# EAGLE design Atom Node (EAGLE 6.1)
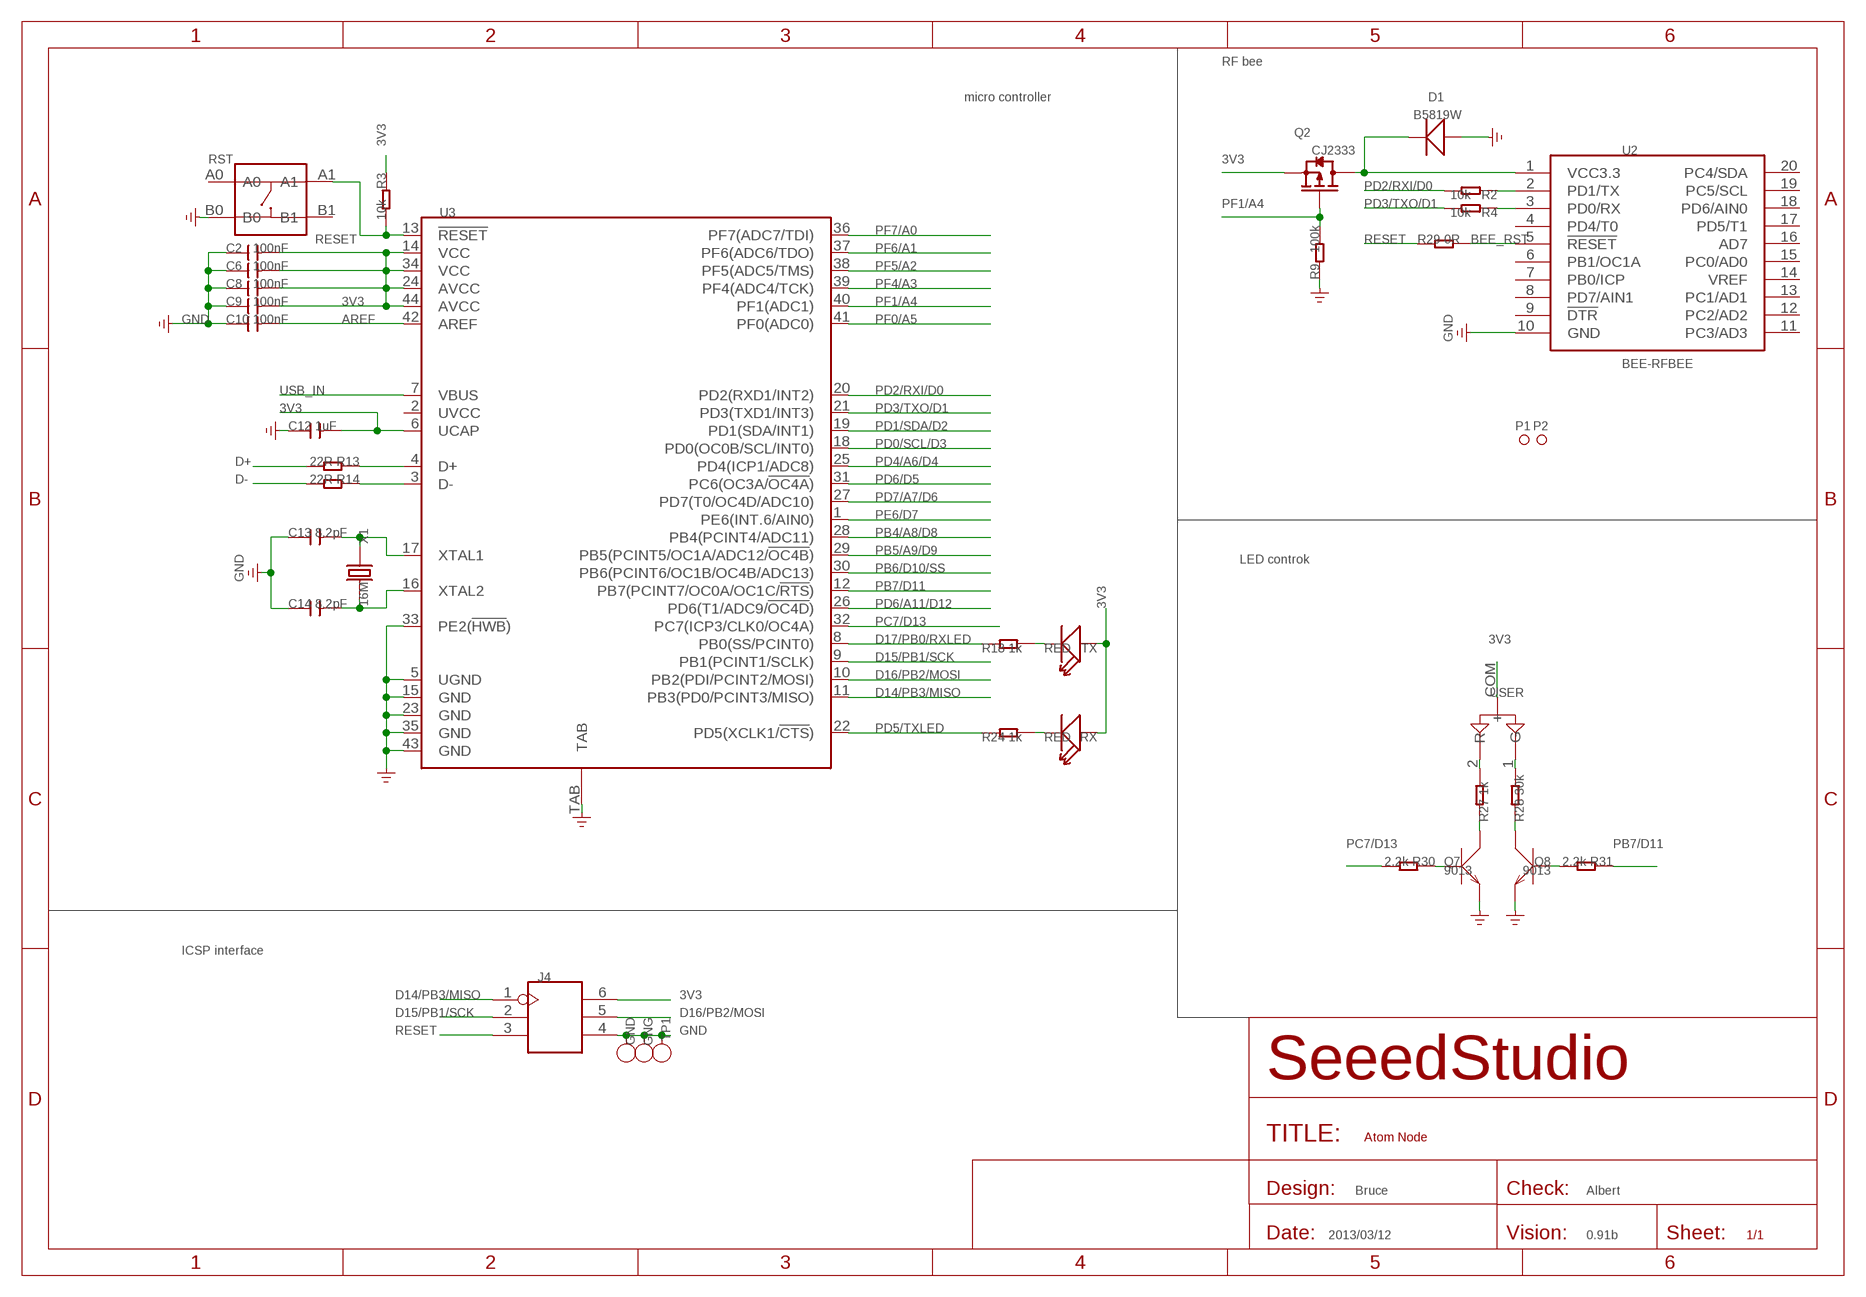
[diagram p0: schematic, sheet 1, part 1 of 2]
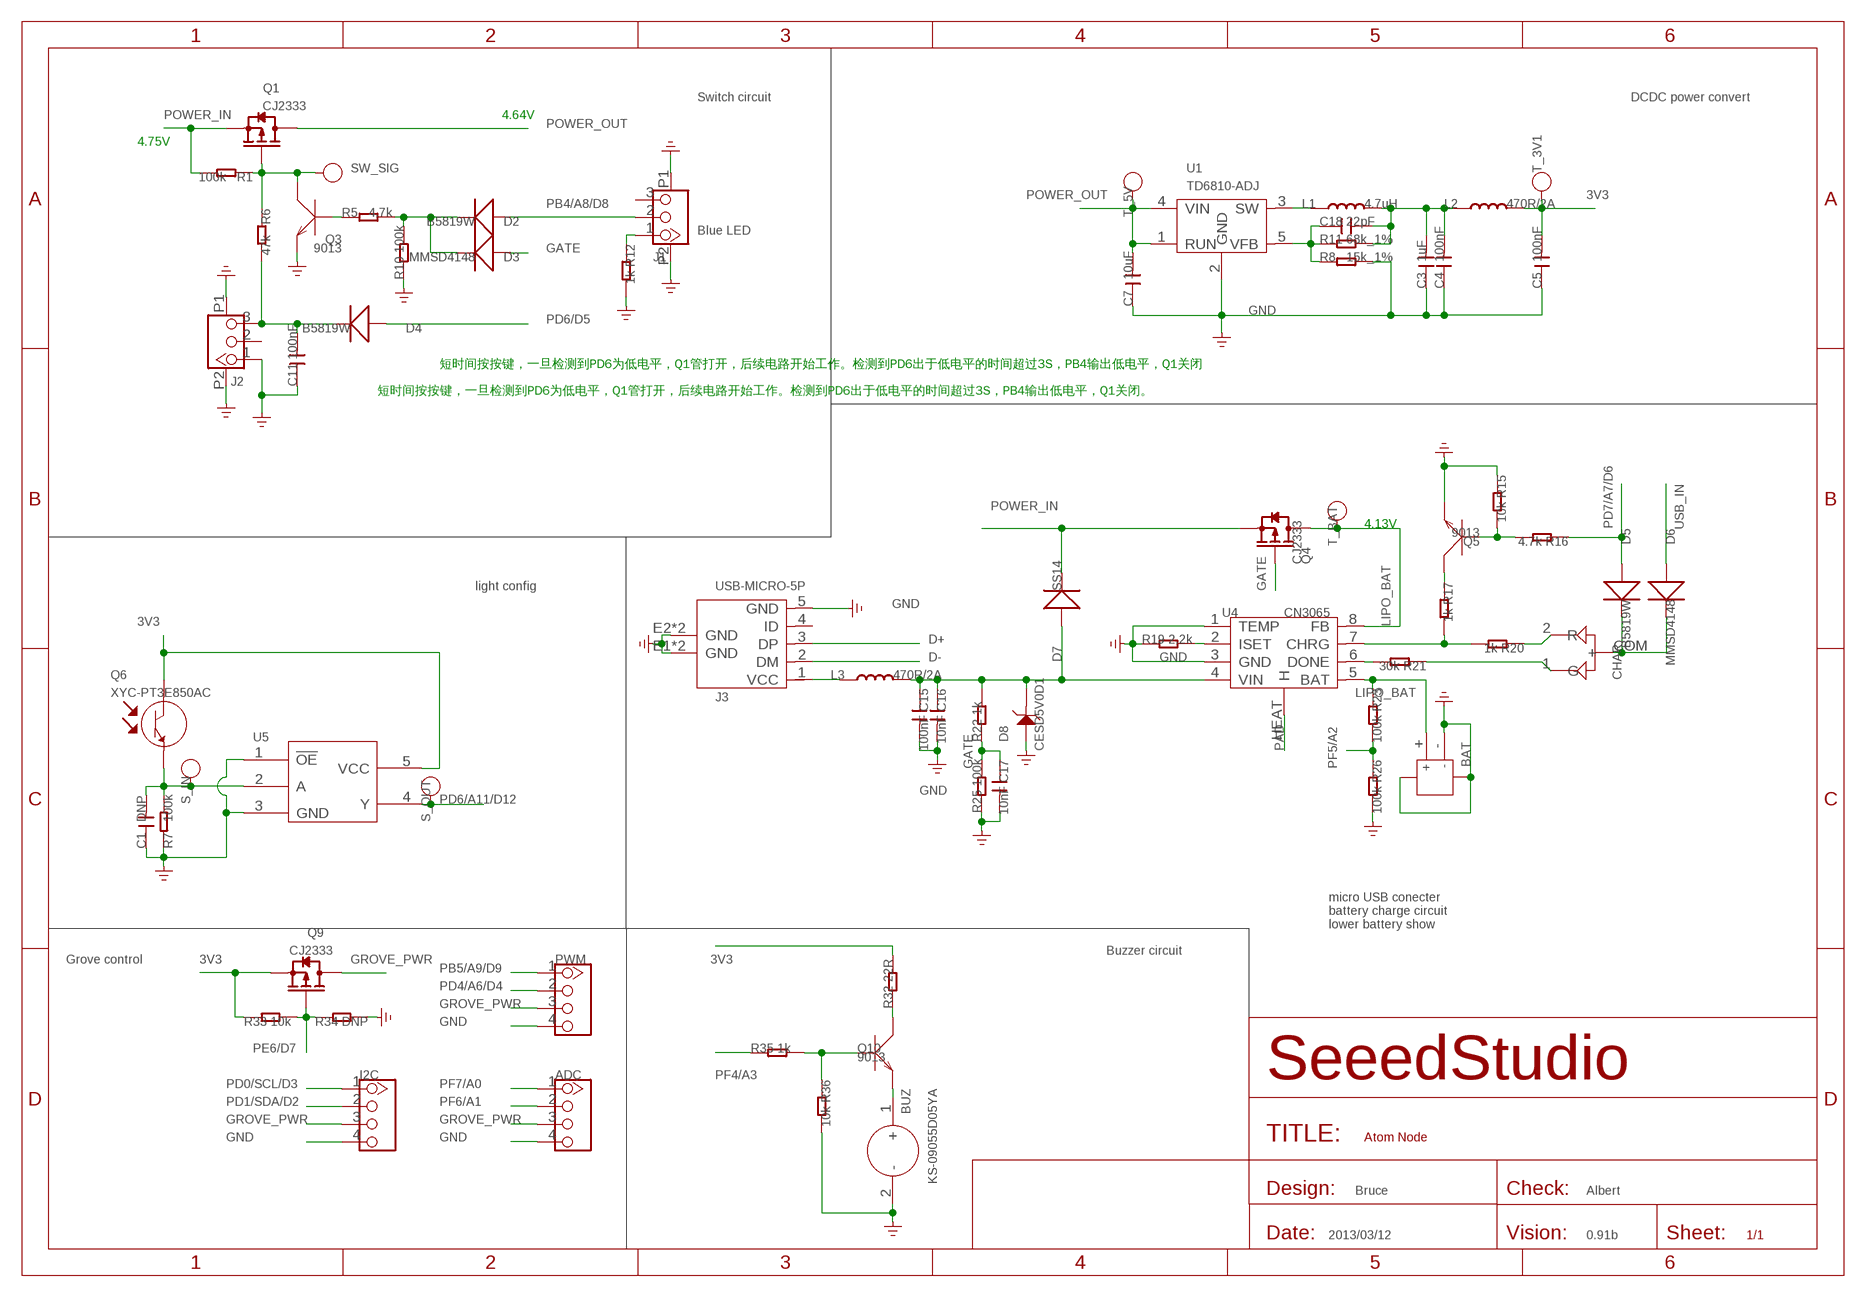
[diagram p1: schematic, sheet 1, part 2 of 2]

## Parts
ADC  TWIG-4P-2.0-2.0  [4P-2.0]
BAT  JACK-JST-2P-SMD-PW'1.0'  [JST-SMD-2P-1.0-90D]
BUZ  KS-09055D05YA  BUZZER-AT0955V5  [2P-5.0-D9.0X5.5H]
C1  DNP  C-0603  [C0603]
C2  100nF  C-0603  [C0603]
C3  1uF  C-0603  [C0603]
C4  100nF  C-0603  [C0603]
C5  100nF  C-0603  [C0603]
C6  100nF  C-0603  [C0603]
C7  10uF  C-0805  [C0805]
C8  100nF  C-0603  [C0603]
C9  100nF  C-0603  [C0603]
C10  100nF  C-0603  [C0603]
C11  100nF  C-0603  [C0603]
C12  1uF  C-0603  [C0603]
C13  8.2pF  C-0603  [C0603]
C14  8.2pF  C-0603  [C0603]
C15  100nF  C-0603  [C0603]
C16  10nF  C-0603  [C0603]
C17  10nF  C-0603  [C0603]
C18  22pF  C-0603  [C0603]
CHAR  LED-ARG-3P'-3MM'  [LED-3P-2.54-3MM]
D1  B5819W  D'1206'  [SOD123]
D2  B5819W  D'1206'  [SOD123]
D3  MMSD4148  D'1206'  [SOD123]
D4  B5819W  D'1206'  [SOD123]
D5  B5819W  D'1206'  [SOD123]
D6  MMSD4148  D'1206'  [SOD123]
D7  SS14  D'B130L-13-F'  [SMA]
D8  CESD5V0D1  D-ESD-2P'CESD5V0D1'  [SOD123-2.7X1.6]
GND  PAD-TEST-POINT-CIRCLE'4545'  [TP_4545]
GNG  PAD-TEST-POINT-CIRCLE'4545'  [TP_4545]
I2C  TWIG-4P-2.0-2.0  [4P-2.0]
J1  JST-3P-1.0  [3P-SMD-1.0]
J2  JST-3P-1.0  [3P-SMD-1.0]
J3  USB-MICRO-5P  [MICRO-USB-5P]
J4  HEADER-2X3P-2.0  [2X3P-2.0]
L1  4.7uH  LSPD3D16-4R7M  [L0420]
L2  470R/2A  L'0805'  [L0805]
L3  470R/2A  L'0805'  [L0805]
P1  PAD-MARK  [ROUND-MARK-1.0]
P2  PAD-MARK  [ROUND-MARK-1.0]
PWM  TWIG-4P-2.0-2.0  [4P-2.0]
Q1  CJ2333  MOSFET-P'SI2323CDS/SI2305DS<BR>'  [SOT23]
Q2  CJ2333  MOSFET-P'SI2323CDS/SI2305DS<BR>'  [SOT23]
Q3  9013  TRANSISTOR-NPN-SOT23  [SOT23]
Q4  CJ2333  MOSFET-P'SI2323CDS/SI2305DS<BR>'  [SOT23]
Q5  9013  TRANSISTOR-NPN-SOT23  [SOT23]
Q6  XYC-PT3E850AC  PHOTISTOR-PT550'XYC-PT3E550AC-IC'  [2P-D3MMX3.85H]
Q7  9013  TRANSISTOR-NPN-SOT23  [SOT23]
Q8  9013  TRANSISTOR-NPN-SOT23  [SOT23]
Q9  CJ2333  MOSFET-P'SI2323CDS/SI2305DS<BR>'  [SOT23]
Q10  9013  TRANSISTOR-NPN-SOT23  [SOT23]
R1  100k  R-0603  [R0603]
R2  10k  R-0603  [R0603]
R3  10k  R-0603  [R0603]
R4  10k  R-0603  [R0603]
R5  4.7k  R-0603  [R0603]
R6  47k  R-0603  [R0603]
R7  100k  R-0603  [R0603]
R8  15k_1%  R-0603  [R0603]
R9  100k  R-0603  [R0603]
R10  100k  R-0603  [R0603]
R11  68k_1%  R-0603  [R0603]
R12  1k  R-0603  [R0603]
R13  22R  R-0603  [R0603]
R14  22R  R-0603  [R0603]
R15  10k  R-0603  [R0603]
R16  4.7k  R-0603  [R0603]
R17  1k  R-0603  [R0603]
R18  1k  R-0603  [R0603]
R19  2.2k  R-0603  [R0603]
R20  1k  R-0603  [R0603]
R21  30k  R-0603  [R0603]
R22  1k  R-0603  [R0603]
R23  100k  R-0603  [R0603]
R24  1k  R-0603  [R0603]
R25  100k  R-0603  [R0603]
R26  100k  R-0603  [R0603]
R27  1k  R-0603  [R0603]
R28  30k  R-0603  [R0603]
R29  0R  R-0603  [R0603]
R30  2.2k  R-0603  [R0603]
R31  2.2k  R-0603  [R0603]
R32  22R  R-0603  [R0603]
R33  10k  R-0603  [R0603]
R34  DNP  R-0603  [R0603]
R35  1k  R-0603  [R0603]
R36  10k  R-0603  [R0603]
RST  BUTTON-4P-3.3X3.3  [4P-SMD-3.4X3.4X1.3H]
RX  RED  LED'0603'  [LED-0603]
S_IN  PAD-TEST-POINT-CIRCLE'4545'  [TP_4545]
S_OUT  PAD-TEST-POINT-CIRCLE'4545'  [TP_4545]
SW_SIG  PAD-TEST-POINT-CIRCLE'4545'  [TP_4545]
T_3V1  PAD-TEST-POINT-CIRCLE'4545'  [TP_4545]
T_5V  PAD-TEST-POINT-CIRCLE'4545'  [TP_4545]
T_BAT  PAD-TEST-POINT-CIRCLE'4545'  [TP_4545]
TP1  PAD-TEST-POINT-CIRCLE'4545'  [TP_4545]
TX  RED  LED'0603'  [LED-0603]
U1  TD6810-ADJ  TD6810'TSOT23-5'  [SOT23-5]
U2  BEE-RFBEE  [20P-DIP-2.0-PRO]
U3  ATMEGA32U4-QFN44  [QFN44]
U4  CN3065  [DFN8]
U5  74AUP1G17GW  SN74LVC1G125DCKR  [SOT353]
USER  LED-ARG-3P'-3MM'  [LED-3P-2.54-3MM]
X1  16M  CRYSTAL'5032'  [2P-SMD-5X3.2]

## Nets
3V3: C2.2 C5.2 C6.2 C8.2 C9.2 C12.2 J4.6 L2.2 Q2.2(S) Q6.C Q9.2(S) R3.1 R32.2 R33.1 RX.+ T_3V1.T TX.+ U3.6(UCAP) U3.14(VCC) U3.24(AVCC) U3.34(VCC) U3.44(AVCC) U5.5(VCC) USER.COM(+)
AREF: C10.2 U3.42(AREF)
BEE_RST: R29.2 U2.5(!RESET)
D14/PB3/MISO: J4.1 U3.11(PB3(PD0/PCINT3/MISO))
D15/PB1/SCK: J4.2 U3.9(PB1(PCINT1/SCLK))
D16/PB2/MOSI: J4.5 U3.10(PB2(PDI/PCINT2/MOSI))
D17/PB0/RXLED: R18.1 U3.8(PB0(SS/PCINT0))
D+: J3.3(DP) R13.2
D-: J3.2(DM) R14.2
GATE: C17.1 D3.+ Q4.1(G) R22.1 R25.2
GND: ADC.4 BAT.3 BAT.4 BAT.- BUZ.2(-) C1.1 C2.1 C3.1 C4.1 C5.1 C6.1 C7.1 C8.1 C9.1 C10.1 C11.1 C12.1 C13.1 C14.1 C15.2 C16.2 C17.2 D1.+ D8.1 GND.T GNG.T I2C.4 J1.P1 J1.P2 J2.1 J2.P1 J2.P2 J3.5(GND) J3.E1(GND) J3.E2(GND) J3.P1(GND) J3.P2(GND) J4.4 PWM.4 Q3.2(E) Q5.2(E) Q7.2(E) Q8.2(E) R7.1 R8.2 R9.1 R10.1 R12.2 R15.1 R19.1 R25.1 R26.2 R34.2 R36.2 RST.B0 TP1.T U1.2(GND) U2.10(GND) U3.5(UGND) U3.15(GND) U3.23(GND) U3.33(PE2(!HWB!)) U3.35(GND) U3.43(GND) U3.TAB U4.1(TEMP) U4.3(GND) U5.1(!OE!) U5.3(GND)
GROVE_PWR: ADC.3 I2C.3 PWM.3 Q9.3(D)
LIPO_BAT: BAT.+ Q4.3(D) R23.1 T_BAT.T U4.5(BAT) U4.8(FB)
N$1: CHAR.COM(+) D5.- D6.-
N$2: Q5.3(C) R17.1
N$3: Q10.3(C) R32.1
N$4: C1.2 Q6.E R7.2 S_IN.T U5.2(A)
N$5: C11.2 D4.- J2.3 R6.2
N$6: BUZ.1(+) Q10.2(E)
N$7: R19.2 U4.2(ISET)
N$8: R17.2 R20.2 U4.7(CHRG)
N$9: R21.2 U4.6(DONE)
N$10: Q1.1(G) Q3.3(C) R1.1 R6.1 SW_SIG.T
N$11: Q10.1(B) R35.2 R36.1
N$12: Q3.1(B) R5.1
N$13: D2.- D3.- R5.2 R10.2
N$14: J3.1(VCC) L3.1
N$15: D1.- Q2.3(D) U2.1(VCC3.3)
N$16: R2.1 U2.2(PD1/TX)
N$17: R4.1 U2.3(PD0/RX)
N$26: Q5.1(B) R15.2 R16.2
N$27: J1.1 R12.1
N$29: L1.1 U1.3(SW)
N$31: C13.2 U3.17(XTAL1) X1.1
N$32: C14.2 U3.16(XTAL2) X1.2
N$33: R18.2 TX.-
N$34: R24.2 RX.-
N$35: Q7.1(B) R30.1
N$37: R13.1 U3.4(D+)
N$38: R14.1 U3.3(D-)
N$39: C18.1 R8.1 R11.1 U1.5(VFB)
N$40: R27.2 USER.2(R)
N$41: CHAR.2(R) R20.1
N$42: CHAR.1(G) R21.1
N$43: R28.2 USER.1(G)
N$44: Q7.3(C) R27.1
N$45: Q8.3(C) R28.1
N$46: Q8.1(B) R31.2
N$47: C3.2 C4.2 C18.2 L1.2 L2.1 R11.2
PAD: U4.HEAT(H)
PB4/A8/D8: D2.+ J1.2 U3.28(PB4(PCINT4/ADC11))
PB5/A9/D9: PWM.1 U3.29(PB5(PCINT5/OC1A/ADC12/!OC4B!))
PB6/D10/SS: U3.30(PB6(PCINT6/OC1B/OC4B/ADC13))
PB7/D11: R31.1 U3.12(PB7(PCINT7/OC0A/OC1C/!RTS!))
PC7/D13: R30.2 U3.32(PC7(ICP3/CLK0/OC4A))
PD0/SCL/D3: I2C.1 U3.18(PD0(OC0B/SCL/INT0))
PD1/SDA/D2: I2C.2 U3.19(PD1(SDA/INT1))
PD2/RXI/D0: R2.2 U3.20(PD2(RXD1/INT2))
PD3/TXO/D1: R4.2 U3.21(PD3(TXD1/INT3))
PD4/A6/D4: PWM.2 U3.25(PD4(ICP1/ADC8))
PD5/TXLED: R24.1 U3.22(PD5(XCLK1/!CTS!))
PD6/A11/D12: S_OUT.T U3.26(PD6(T1/ADC9/!OC4D!)) U5.4(Y)
PD6/D5: D4.+ U3.31(PC6(OC3A/!OC4A!))
PD7/A7/D6: D5.+ R16.1 U3.27(PD7(T0/OC4D/ADC10))
PE6/D7: Q9.1(G) R33.2 R34.1 U3.1(PE6(INT.6/AIN0))
PF0/A5: U3.41(PF0(ADC0))
PF1/A4: Q2.1(G) R9.2 U3.40(PF1(ADC1))
PF4/A3: R35.1 U3.39(PF4(ADC4/TCK))
PF5/A2: R23.2 R26.1 U3.38(PF5(ADC5/TMS))
PF6/A1: ADC.2 U3.37(PF6(ADC6/TDO))
PF7/A0: ADC.1 U3.36(PF7(ADC7/TDI))
POWER_IN: D7.1(-) Q1.2(S) Q4.2(S) R1.2
POWER_OUT: C7.2 Q1.3(D) T_5V.T U1.1(RUN) U1.4(VIN)
RESET: J4.3 R3.2 R29.1 RST.A1 U3.13(!RESET)
USB_IN: C15.1 C16.1 D6.+ D7.2(+) D8.2 L3.2 R22.2 U3.7(VBUS) U4.4(VIN)
Unconnected: J1.3 J2.2 J3.4(ID) RST.A0 RST.B1 U2.4(PD4/T0) U2.6(PB1/OC1A) U2.7(PB0/ICP) U2.8(PD7/AIN1) U2.9(!DTR) U2.11(PC3/AD3) U2.12(PC2/AD2) U2.13(PC1/AD1) U2.14(VREF) U2.15(PC0/AD0) U2.16(AD7) U2.17(PD5/T1) U2.18(PD6/AIN0) U2.19(PC5/SCL) U2.20(PC4/SDA) U3.2(UVCC)

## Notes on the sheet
- RF bee
- micro controller | Switch circuit | DCDC power convert
- 4.64V
- 4.75V
- Blue LED
- 短时间按按键，一旦检测到PD6为低电平，Q1管打开，后续电路开始工作。检测到PD6出于低电平的时间超过3S，PB4输出低电平，Q1关闭
- 短时间按按键，一旦检测到PD6为低电平，Q1管打开，后续电路开始工作。检测到PD6出于低电平的时间超过3S，PB4输出低电平，Q1关闭。
- 4.13V
- LED controk
- light config
- micro USB conecter
  battery charge circuit
  lower battery show
- ICSP interface | Buzzer circuit
- Grove control
- Bruce | Albert | Bruce | Albert
- 2013/03/12 | 0.91b | 2013/03/12 | 0.91b

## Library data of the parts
ADC I2C PWM = Connector:TWIG-4P-2.0
BAT = Connector:JACK-JST-2P-SMD-PW
BUZ = Discrete:BUZZER
C1-C18 = Discrete:C*: Ceramic Capacitors
CHAR USER = Discrete:LED-ARG-3P
D1-D7 = Discrete:D*
D8 = Discrete:D-ESD-2P: Diodes for Protectiong against ESD
GND GNG S_IN S_OUT SW_SIG T_3V1 T_5V T_BAT TP1 = Discrete:PAD-TEST-POINT-CIRCLE; PARTNO: DNP
J1 J2 = template:JST-3P-1.0
J3 = Connector:USB-MICRO-5P
J4 = Connector:HEADER-2X3P
L1 = template:L
L2 L3 = Discrete:L*
P1 P2 = Discrete:PAD-MARK; PARTNO: DNP
Q1 Q2 Q4 Q9 = Discrete:MOSFET-P
Q3 Q5 Q7 Q8 Q10 = Discrete:TRANSISTOR-NPN*: NPN audion
Q6 = template:PHOTISTOR-PT550
R1-R36 = Discrete:R*
RST = Discrete:BUTTON-4P
RX TX = Discrete:LED*
U1 = template:TD6810: 1.5MHz 800mA Synchronous Step-Down Regulator Dropout http://www.techcodeok.com/download/TD6810.pdf
U2 = moudle:BEE-RFBEE
U3 = IC:ATMEGA32U4-QFN44: 8-bit Microcontroller With 16/32K Bytes of ISP Flash and USB controller
U4 = IC:CN3065
U5 = template:SN74LVC1G125DCKR: Signal bus buffer gate
X1 = Discrete:CRYSTAL*: CRYSTAL

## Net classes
0 default: width 0.152 mm, drill 0.305 mm, clearance 0.152 mm
3 none3: width 0.203 mm, drill 0.305 mm, clearance 0.203 mm

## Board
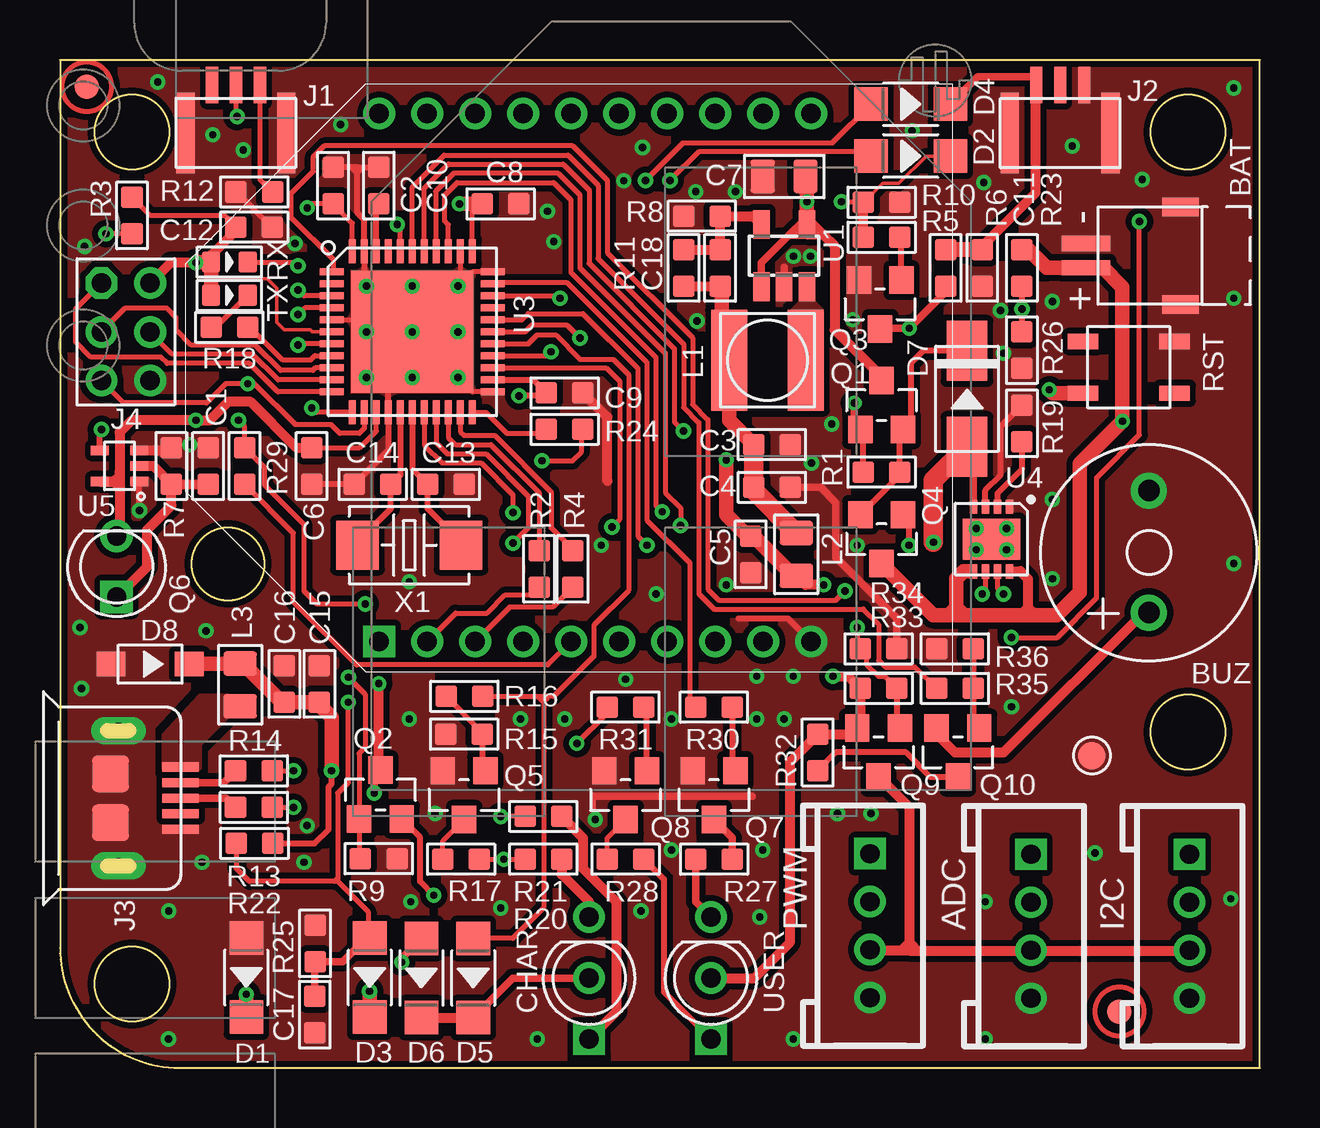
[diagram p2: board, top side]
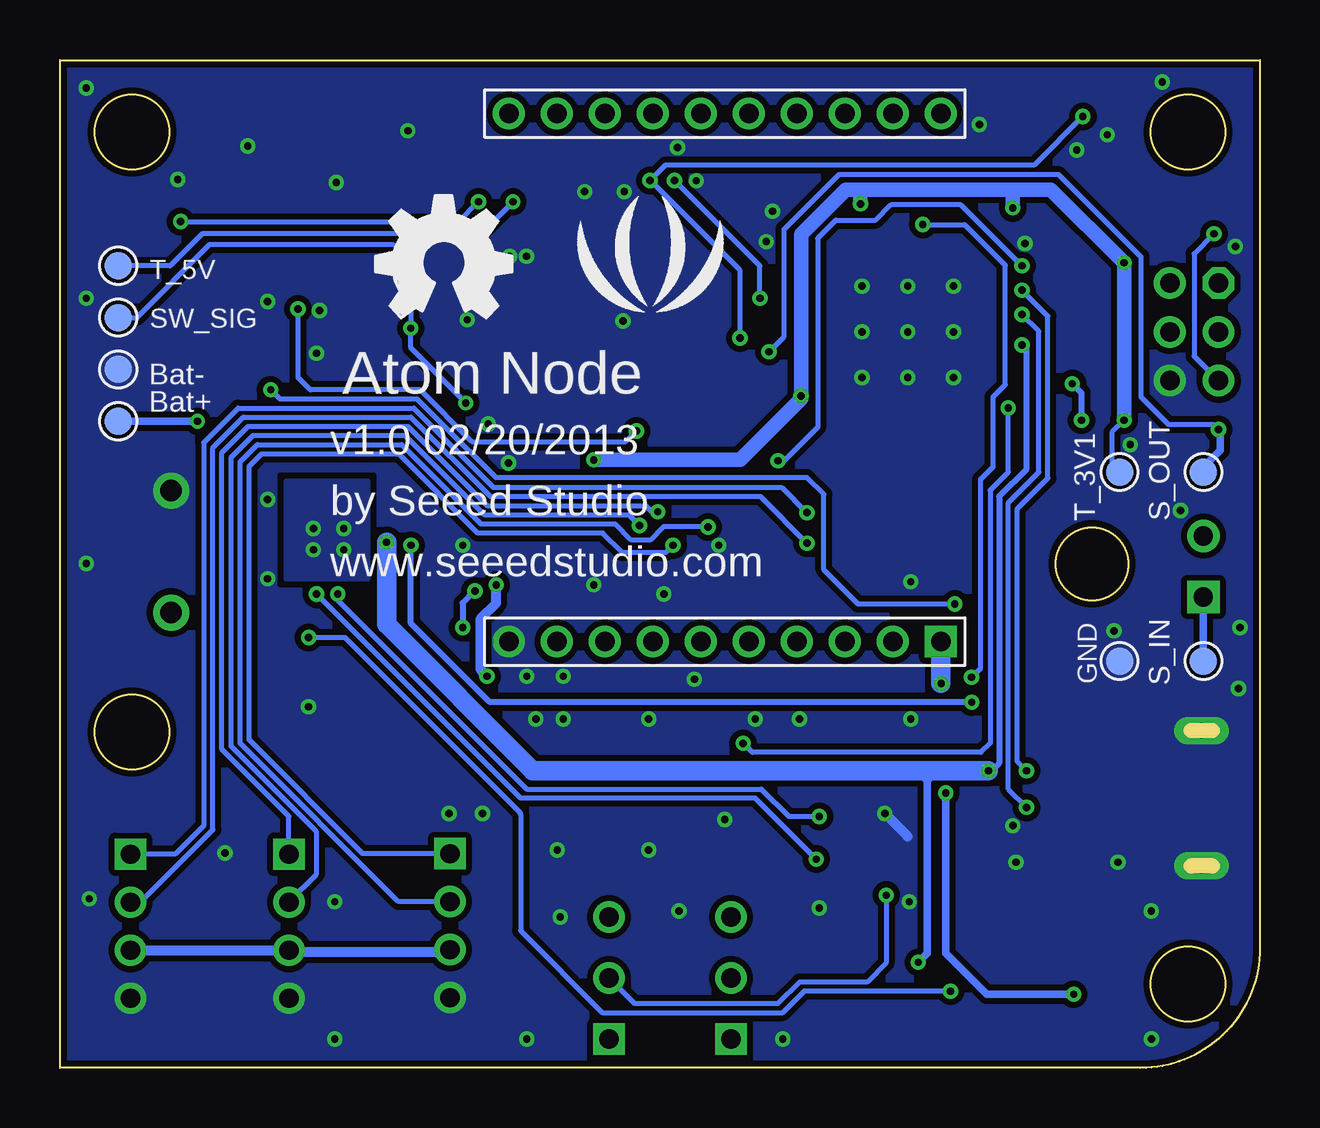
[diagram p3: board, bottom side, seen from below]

Size 50 x 42 mm. Coordinates in mm from the lower left corner, seen from the top.
Outline: 5,0 4.76,0 4.52,0.02 4.29,0.05 4.05,0.09 3.82,0.14 3.59,0.2 3.36,0.27 3.14,0.36 2.92,0.45 2.71,0.56 2.5,0.67 2.3,0.79 2.1,0.93 1.91,1.07 1.72,1.22 1.55,1.38 1.38,1.55 1.22,1.72 1.07,1.91 0.93,2.1 0.79,2.3 0.67,2.5 0.56,2.71 0.45,2.92 0.36,3.14 0.27,3.36 0.2,3.59 0.14,3.82 0.09,4.05 0.05,4.29 0.02,4.52 0.01,4.76 0,5 0,42 50,42 50,0 5,0
Outline: circle at 3,39 radius 1.55
Outline: circle at 7,21 radius 1.52
Outline: circle at 47,39 radius 1.55
Outline: circle at 3,3.5 radius 1.55
Outline: circle at 47,14 radius 1.55
Copper layers (1*16): Top 0.035mm / dielectric 1.5mm / Bottom 0.035mm
Design rules "SeeedStudio_rule_no_angle_090911 *": minimum track width 6mil, minimum drill 12mil, track to track 6mil, track to pad 6mil, pad to pad 6mil, via to via 6mil, smd to smd 0mil, copper to edge 8mil, drill to drill 10mil, minimum pad ring 10mil, minimum via ring 6mil, stop-mask expansion 2mil, vias tented up to drill 25mil, thermal gap 10mil
tRestrict: area 28,27.4 to 30.9,31.4

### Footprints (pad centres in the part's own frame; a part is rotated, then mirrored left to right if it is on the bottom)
4P-2.0 = drill 0.8 pad 1.27 square: 1 -3,0 | drill 0.8 pad 1.27: 2 -1,0; 3 1,0; 4 3,0
JST-SMD-2P-1.0-90D = smd 1.524 x 0.762: 3 -3.429,2.032; 4 -3.429,-2.032 | smd 2.032 x 0.635: + 0.508,0.508; - 0.508,-0.508
2P-5.0-D9.0X5.5H = drill 0.9 pad 1.5: 1 -2.5,0; 2 2.58,0
C0603 = smd 0.889 x 0.889: 1 -0.762,0; 2 0.762,0
C0805 = smd 1.016 x 1.397: 1 -0.889,0; 2 0.889,0
LED-3P-2.54-3MM = drill 0.8 pad 1.3 square: 1 -2.54,0 | drill 0.8 pad 1.3: 2 2.54,0; COM 0,0
SOD123 = smd 1.397 x 1.397: + -1.651,0; - 1.651,0
SMA = smd 2.5 x 1.7: 1 2,0; 2 -2,0
SOD123-2.7X1.6 = smd 1.2 x 1.02: 1 -1.635,0; 2 1.635,0
TP_4545 = smd 1.143 x 1.143: T 0,0
3P-SMD-1.0 = smd 1.524 x 0.508: 1 -2,1; 2 -2,0; 3 -2,-1 | smd 3.353 x 0.762: P1 0,-2.1; P2 0,2.1
MICRO-USB-5P = smd 0.38 x 1.52: 1 -1.3,0; 2 -0.65,0; 3 0,0; 4 0.65,0; 5 1.3,0 | smd 1.524 x 1.524: E1 -1.016,-2.921; E2 1.016,-2.921 | drill 0.635 pad 1.143 long: P1 -2.819,-2.591; P2 2.819,-2.591
2X3P-2.0 = drill 0.813 pad 1.27 octagon: 1 -1.016,2.032 | drill 0.813 pad 1.27: 2 -1.016,0; 3 -1.016,-2.032; 4 1.016,-2.032; 5 1.016,0; 6 1.016,2.032
L0420 = smd 1.5 x 4.2: 1 -1.6,0; 2 1.6,0
L0805 = smd 1.016 x 1.397: 1 -0.889,0; 2 0.889,0
ROUND-MARK-1.0 = smd 1.016 x 1.016: P$1 0,0
SOT23 = smd 1.016 x 1.143: 1 -0.889,-1.016; 2 0.889,-1.016; 3 0,1.016
2P-D3MMX3.85H = drill 0.8 pad 1.35: C 1.27,0 | drill 0.8 pad 1.35 square: E -1.27,0
R0603 = smd 0.889 x 0.889: 1 -0.762,0; 2 0.762,0
4P-SMD-3.4X3.4X1.3H = smd 1.27 x 0.635: A0 -1.905,1.079; A1 1.905,1.079; B0 -1.905,-1.079; B1 1.905,-1.079
LED-0603 = smd 0.762 x 0.889: + -0.762,0; - 0.762,0
SOT23-5 = smd 0.69 x 1.2: 1 -0.95,-1.3; 2 0,-1.3; 3 0.95,-1.3; 4 0.95,1.3; 5 -0.95,1.3
20P-DIP-2.0-PRO = drill 0.813 square: 1 -11,9 | drill 0.813: 2 -11,7; 3 -11,5; 4 -11,3; 5 -11,1; 6 -11,-1; 7 -11,-3; 8 -11,-5; 9 -11,-7; 10 -11,-9; 11 11,-9; 12 11,-7; 13 11,-5; 14 11,-3; 15 11,-1; 16 11,1; 17 11,3; 18 11,5; 19 11,7; 20 11,9
QFN44 = smd 1 x 0.3: 1 -3.35,2.5; 2 -3.35,2; 3 -3.35,1.5; 4 -3.35,1; 5 -3.35,0.5; 6 -3.35,0; 7 -3.35,-0.5; 8 -3.35,-1; 9 -3.35,-1.5; 10 -3.35,-2; 11 -3.35,-2.5; 23 3.35,-2.5; 24 3.35,-2; 25 3.35,-1.5; 26 3.35,-1; 27 3.35,-0.5; 28 3.35,0; 29 3.35,0.5; 30 3.35,1; 31 3.35,1.5; 32 3.35,2; 33 3.35,2.5 | smd 0.3 x 1: 12 -2.5,-3.35; 13 -2,-3.35; 14 -1.5,-3.35; 15 -1,-3.35; 16 -0.5,-3.35; 17 0,-3.35; 18 0.5,-3.35; 19 1,-3.35; 20 1.5,-3.35; 21 2,-3.35; 22 2.5,-3.35; 34 2.5,3.35; 35 2,3.35; 36 1.5,3.35; 37 1,3.35; 38 0.5,3.35; 39 0,3.35; 40 -0.5,3.35; 41 -1,3.35; 42 -1.5,3.35; 43 -2,3.35; 44 -2.5,3.35 | smd 5.08 x 5.08: TAB 0,0
DFN8 = smd 0.3 x 0.6: 1 -0.75,-1.35; 2 -0.25,-1.35; 3 0.25,-1.35; 4 0.75,-1.35; 5 0.75,1.35; 6 0.25,1.35; 7 -0.25,1.35; 8 -0.75,1.35 | smd 2.4 x 1.7: HEAT 0,0
SOT353 = smd 0.4 x 0.75: 1 -0.65,-0.825; 2 0,-0.825; 3 0.65,-0.825; 4 0.65,0.825; 5 -0.65,0.825
2P-SMD-5X3.2 = smd 1.778 x 2.032: 1 -2.159,0; 2 2.159,0

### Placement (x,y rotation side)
ADC  40.46,5.91 270 top
BAT  43.25,33.85 180 top
BUZ  45.37,21.48 90 top
C1  6.17,25.08 270 top
C2  11.38,36.77 270 top
C3  29.66,25.97 180 top
C4  29.66,24.19 180 top
C5  28.78,21.4 90 top
C6  10.49,25.08 90 top
C7  30.17,37.15 0 top
C8  18.36,36.01 180 top
C9  21.03,28.13 180 top
C10  13.28,36.77 270 top
C11  38.43,33.34 90 top
C12  8.09,35.04 180 top
C13  16.08,24.32 180 top
C14  13.03,24.32 0 top
C15  10.8,16 90 top
C16  9.34,16 90 top
C17  10.61,2.22 270 top
C18  27.51,33.34 270 top
CHAR  22.04,3.75 90 top
D1  7.76,3.77 270 top
D2  35.45,38 0 top
D3  12.91,3.77 270 top
D4  35.45,40.16 0 top
D5  17.22,3.75 270 top
D6  15.06,3.75 270 top
D7  37.79,27.88 90 top
D8  3.76,16.83 0 top
GND  5.85,16.96 90 bottom
GNG  43,13.02 270 top
I2C  47.06,5.91 270 top
J1  7.33,38.96 270 top
J2  41.67,38.95 270 top
J3  5.03,11.24 270 top
J4  2.74,30.67 0 top
L1  29.48,29.49 180 top
L2  30.68,21.4 270 top
L3  7.51,15.96 90 top
P1  1.11,40.88 270 top
P2  44.14,2.35 270 top
PWM  33.75,5.93 270 top
Q1  34.24,27.62 0 top
Q2  13.35,11.39 0 top
Q3  34.17,31.81 180 top
Q4  34.24,22.04 180 top
Q5  16.84,11.37 180 top
Q6  2.36,20.89 90 top
Q7  27.25,11.37 180 top
Q8  23.57,11.37 180 top
Q9  34.11,13.15 180 top
Q10  37.41,13.15 180 top
R1  34.24,24.83 0 top
R2  19.96,20.79 90 top
R3  3,35.52 270 top
R4  21.36,20.79 90 top
R5  34.24,34.61 180 top
R6  36.9,33.34 90 top
R7  4.65,25.08 270 top
R8  26.74,35.5 180 top
R9  13.28,8.72 180 top
R10  34.24,36.07 180 top
R11  25.98,33.34 270 top
R12  8.09,36.5 180 top
R13  8.07,10.86 180 top
R14  8.07,12.38 180 top
R15  16.84,13.91 0 top
R16  16.85,15.48 180 top
R17  16.71,8.7 0 top
R18  7.06,30.86 180 top
R19  40.08,26.86 270 top
R20  20.14,8.7 180 top
R21  20.14,10.48 180 top
R22  8.1,9.35 0 top
R23  40.08,33.34 270 top
R24  21.03,26.61 0 top
R25  10.63,5.19 270 top
R26  40.08,29.91 270 top
R27  27.25,8.7 180 top
R28  23.57,8.7 0 top
R29  7.69,25.08 270 top
R30  27.24,15.04 180 top
R31  23.56,15.04 0 top
R32  31.57,13.15 90 top
R33  34.11,15.81 0 top
R34  34.11,17.46 0 top
R35  37.28,15.81 0 top
R36  37.28,17.46 180 top
RST  44.53,29.2 180 top
RX  7.06,33.58 0 top
S_IN  2.36,16.96 90 bottom
S_OUT  2.36,24.83 90 bottom
SW_SIG  47.57,31.27 90 bottom
T_3V1  5.85,24.83 90 bottom
T_5V  47.57,33.43 90 bottom
T_BAT  47.57,26.95 180 bottom
TP1  47.57,29.11 90 bottom
TX  7.06,32.2 0 top
U1  30.17,33.85 0 top
U2  22.3,28.77 90 top
U3  14.68,30.67 0 top
U4  38.81,22.04 180 top
U5  2.49,25.08 90 top
U$4  [LOGO_SILK]  25.42,33.17 0 bottom
U$13  [OSHW_FILLX200_NOTEXT]  36.85,31.27 0 bottom
USER  27.12,3.75 90 top
X1  14.55,21.78 180 top

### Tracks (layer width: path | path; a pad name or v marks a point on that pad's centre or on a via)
3V3  (via drill 0.3 pad 0.64)
  Top 0.152: U3.6 10.52,30.67 10.43,30.76 9.34,30.76 9.03,31.08 9.03,32.5 8.64,32.88 6.3,32.88
  Top 0.203: C6.2 12.49,25.85 13.18,26.54 U3.14 | U3.44 12.18,35.2 C2.2 10.47,36.01 v10.3,35.84 | 2.1,24.43 2.1,24.44 2.49,24.83 | U3.34 17.18,36.01 C8.2 | R3.1 3.76,35.52 6.84,35.52 C12.2
  Top 0.254: U3.24 19.73,28.67 C9.2 20.14,28 v19.12,28 | v15.57,7.2 15,7.77 15,9.61 Q2.2
  Top 0.406: v32.2,16.32 32.84,16.32 R33.1 33.35,14.06 33.42,13.99 33.39,13.99 Q9.2 32.97,13.91 R32.2 30.43,12.76 30.43,5.24 28.93,3.75 USER.COM | 2.49,24.45 2.49,24.83 2.49,26.48 2.99,26.99 v5.66,26.99 6.24,26.99 7,27.75 7.95,27.75 9.85,25.85 C6.2 | 2.49,24.45 2.49,24.19 | 2.49,24.19 2.49,22.29 Q6.C | U5.5 2.1,24.43 2.25,24.43 | 2.25,24.43 2.47,24.43 2.49,24.45 | v31.82,20.13 31.06,20.13 L2.2 | 2.25,24.43 2.49,24.19 | v5.66,33.55 4.61,33.55 J4.6 | RX.+ 6.3,33.86 7.32,34.89 C12.2
  Top 0.61: v16.65,36.01 C8.2 | L2.2 30.55,20.51 28.9,22.16 C5.2 28.65,22.16 27.76,23.05 v27.76,25.34 | TX.+ 6.3,32.88 RX.+ 5.69,33.58 v5.66,33.55
  Bottom 0.203: v5.66,26.99 6.17,26.48 6.17,25.15 T_3V1.T | 10.3,36.47 10.43,36.6 | USER.COM 26.07,2.69 20.08,2.69 19.19,3.58 16.37,3.58 15.57,4.38 v15.57,7.2
  Bottom 0.406: v32.2,16.32 32.46,16.57 32.46,18.73 31.82,19.37 v31.82,20.13
  Bottom 0.61: 16.78,36.6 10.43,36.6 8.71,36.6 v5.66,33.55 v5.66,26.99 | 16.78,36.6 17.26,36.6 19.12,34.74 v19.12,28 19.12,27.88 21.66,25.34 v27.76,25.34 | v10.3,35.84 10.3,36.47 | v16.65,36.01 16.65,36.47 16.78,36.6
AREF
  Top 0.254: U3.42 13.18,35.9 C10.2
BEE_RST
  Top 0.203: U2.5 20.33,16.8 12.36,16.8 9.73,19.43 9.73,22.29 R29.2
D14/PB3/MISO
  Top 0.203: J4.1 0.65,31.63 0.65,30.25 1.29,29.62 4.21,29.62 4.46,29.36 7.89,29.36 9.08,28.17 U3.11
D15/PB1/SCK
  Top 0.203: U3.9 10.64,29.17 10.54,29.07 9.2,29.07 8.14,30.12 5.48,30.12 4.84,30.76 4.84,31.27 4.46,31.65 2.7,31.65 J4.2
D16/PB2/MOSI
  Top 0.203: U3.10 9.09,28.67 8.02,29.74 4.69,29.74 J4.5
D17/PB0/RXLED
  Top 0.203: R18.1 8.04,30.86 8.02,30.84 8.02,30.76 | U3.8 11.32,29.68 10.62,29.68 10.43,29.49 9.29,29.49 8.02,30.76 | 8.02,30.76 8.14,30.76
D+
  Top 0.305: J3.3 6.93,11.24 R13.2
D-
  Top 0.305: J3.2 6.82,11.89 R14.2
GATE  (via drill 0.3 pad 0.64)
  Top 0.203: v12.01,15.24 12.01,11.89 11.57,11.45 11.57,7.9 | 11.57,7.9 11.57,7.77 | 11.57,7.77 12.84,6.5 12.84,5.49 D3.+ | 11.57,7.77 11.45,7.77 | 11.45,7.77 7.89,7.77 7.34,8.32 R22.1 | 11.45,7.77 11.57,7.9
  Top 0.254: v35.38,21.78 35.38,22.8 Q4.1
  Top 0.305: C17.1 R25.2 11.79,4.43 12.84,5.49
  Bottom 0.254: v35.38,21.78 35.38,18.52 32.12,15.26 12.04,15.26 v12.01,15.24
GND  (via drill 0.3 pad 0.64)
  Top 0.203: U3.33 17.18,33.17 v16.58,32.58 16.68,32.67 U3.35 | U3.23 17.18,28.17 v16.58,28.77 | U3.5 12.27,31.17 v12.77,30.67 | R12.2 7.36,36.5 8.65,35.2 | v22.3,10.35 22.24,10.35 22.24,11.33
  Top 0.254: 12.39,37.29 12.39,35.62 12.68,35.34 U3.43 12.68,32.67 v12.77,32.58 | 12.39,37.3 12.39,37.53 | 12.39,37.53 C10.1 | 12.39,37.53 C2.1 | v12.77,28.77 13.66,28.77 13.68,28.75 U3.15 13.68,25.73 C14.1 C6.1 | 28.27,18.73 30.33,18.73 U2.10 | U4.3 38.56,24.07 39.19,24.7 39.19,26.73 R19.1 | v3.31,23.23 3.31,24.38 | 12.39,37.29 12.39,37.3 | 12.39,37.3 12.21,37.49 | 12.39,37.29 12.59,37.49
  Top 0.305: R34.2 34.87,18.73 32.33,21.27 32.33,23.56 31.7,24.19 C4.1 | 22.24,11.33 28.84,11.33 | U1.2 30.17,33.36
  Top 0.406: U5.3 4.53,25.73 R7.1 | 22.81,24.45 22.81,27.12 C9.1
  Bottom 0.406: 14.68,9.65 v15.63,10.61
  other vias: 20.32,35.7 27.76,20.13 14.68,30.67 14.68,32.58 14.68,28.77 16.58,30.67 33.22,21.78 30.55,16.32 23.57,16.19 21.03,14.54 25.47,9.08 32.39,10.61 14.55,14.54 5.41,25.97 28.14,36.51 32.15,26.84 41.35,31.94 45.09,37.02 19.19,14.54 25.47,14.54 29.03,16.32 29.03,14.54 29.28,9.08 29.16,6.29 31.32,25.21 39.19,31.56 39.32,29.78 41.35,23.69 41.35,20.38 33.03,31.18 38.49,36.89 0.9,15.81 18.36,6.67 11.69,39.31 6.08,18.21 19.89,1.21 4.52,1.21 5.92,8.57 0.84,18.35 35.51,39.05 39.65,15.05 43.13,8.95 38.55,6.92 26.49,36.51 1.03,34.23 30.17,14.54 33.79,10.61 30.55,1.21 38.55,1.21 4.53,6.54 48.9,40.83 48.9,32.07 48.9,21.02 48.78,7.05 4.07,41.09 30.57,33.82 14.61,6.92 6.37,38.89 9.79,34.35 7.64,38.25 24.27,38.35 42.17,38.42 24.84,19.75 22.55,21.78 14.55,20.26 24.2,6.54 23.49,36.97 26.54,31.13 10.17,8.57 10.3,10.1 20.57,34.43 31.26,33.82
  pour Bottom (isolate 0.254, rank 6, no thermals): 50.24,42.1 50.24,-0.44 -1.2,-0.44 -1.2,42.1
  pour Top (isolate 0.254, rank 6, no thermals): 50.24,42.1 50.24,-0.44 -1.2,-0.44 -1.2,42.1
GROVE_PWR
  Top 0.305: 35.38,5.23 35.32,5.23 34.94,4.85 35.83,4.85 35.45,5.23
  Top 0.406: Q9.3 35.38,10.86 35.38,5.23 35.38,4.89 | 35.38,4.89 33.8,4.89 PWM.3 | 35.38,4.89 40.44,4.89 | 40.44,4.89 ADC.3 | 40.44,4.89 47.05,4.89 I2C.3
  Bottom 0.406: I2C.3 40.52,4.91 40.46,4.85 33.86,4.85 33.73,4.98
LIPO_BAT  (via drill 0.3)
  Top 0.254: U4.8 39.62,20.69 39.63,20.7 | U4.5 37.81,20.69 37.79,20.7
  Top 0.406: 40.46,18.86 40.33,18.99 40.33,19.18 | 39.63,20.7 40.01,20.7 40.33,20.38 40.33,19.18 | 40.33,19.18 40.59,18.92 | 40.33,19.18 40.08,18.92
  Top 0.61: 37.41,18.86 36.39,18.86 Q4.3 | 37.41,18.86 40.46,18.86 41.53,18.86 42.49,19.83 42.49,25.17 v44.27,26.95 44.27,32.53 43.47,33.34 BAT.+ 41.12,33.34 40.36,34.1 R23.1 | 37.35,19.18 37.35,20.38 37.67,20.7 37.79,20.7 37.92,20.7 | 37.35,19.18 37.35,18.93 37.41,18.86 | 37.35,19.18 37.6,18.92 | 37.35,19.18 37.09,18.92
  Bottom 0.305: T_BAT.T v44.27,26.95
N$1
  Top 0.305: D5.- 18.87,3.75 CHAR.COM
  Top 0.406: D6.- D5.-
N$2
  Top 0.203: R17.1 15.95,9.46 Q5.3
N$3
  Top 0.254: Q10.3 36.27,12.13 35.25,13.15 32.33,13.15 R32.1
N$4
  Top 0.406: U5.2 3.88,25.08 R7.2 | R7.2 C1.2 | Q6.E 3.63,20.89 3.63,22.42 4.65,23.43 R7.2
  Bottom 0.305: S_IN.T Q6.E
N$5
  Top 0.203: 36.78,34.23 R6.2 | 36.97,40.03 37.1,40.03 D4.- | 40.66,41.3 40.67,41.3 J2.3 40.66,40.95 40.66,40.74
  Top 0.305: 40.66,41.3 38.24,41.3 D4.- | 37.1,40.03 37.11,40.04
  Top 0.406: 36.78,34.23 38.41,34.23 40.66,36.47 40.66,40.74
  Top 0.61: R6.2 C11.2
N$6
  Top 0.406: BUZ.1 45.15,18.98 39.32,13.15 37.28,13.15 36.52,13.91 Q10.2
N$7
  Top 0.254: R19.2 40.08,24.96 39.06,23.94 U4.2
N$8  (via drill 0.3 pad 0.64)
  Top 0.203: R17.2 v18.49,8.7 R20.2 | U4.7 39.06,20.01 v39.32,19.75
  Bottom 0.203: 39.32,19.5 v39.32,19.75 30.81,11.24 21.03,11.24 v18.49,8.7
N$9  (via drill 0.3 pad 0.64)
  Top 0.203: R21.2 v18.36,10.48 | U4.6 38.56,19.88 v38.43,19.75
  Bottom 0.203: v38.43,19.75 38.43,19.5 30.55,11.62 20.77,11.62 19.63,10.48 v18.36,10.48
N$10  (via drill 0.3, 0.3 pad 0.64)
  Top 0.203: 34.2,30.82 Q3.3
  Top 0.254: R1.1 33.47,26.48 Q1.1 33.15,26.8 33.09,26.8
  Top 0.305: 36.9,32.54 R6.1 36.78,32.45 36.78,32.22 v35.38,30.82 34.2,30.82 | v33.09,27.71 33.09,26.8
  Bottom 0.203: v33.09,27.71 35.38,30 v35.38,30.82 v35.38,30.83 35.38,33.57 36.12,34.31 43.76,34.31 46.81,31.27 SW_SIG.T
N$11
  Top 0.254: R36.1 R35.2 38.05,14.42 Q10.1
N$12
  Top 0.254: Q3.1 35.06,34.54 R5.1
  Top 0.305: R5.1 35.12,34.48
N$13  (via drill 0.3 pad 0.64)
  Top 0.152: R10.2 33.5,36.07 34.29,36.85 34.94,36.85 36.08,38 D2.-
  Top 0.203: v44.97,35.27 44.97,26.38 43.2,24.6 43.2,19.58 41.54,17.93 v39.64,17.93 | R10.2 32.59,36.07 v32.57,36.09 | 12.84,2.06 D3.- | 12.59,2.44 D3.- | D3.-
  Top 0.254: 32.53,36.09 v32.57,36.09
  Top 0.406: R5.2 R10.2
  Top 0.61: v12.9,3.2 D3.-
  Bottom 0.203: v39.64,17.93 38.12,17.93 30.81,10.63 30.81,10.57 30.81,5.72 27.4,2.31 19.89,2.31 19,3.2 v12.9,3.2 | v32.57,36.09 33.39,35.27 v44.97,35.27
N$14
  pour Top (no thermals): 4.33,12.47 4.33,13.87 5.86,15.52 7,15.52 7,14.69 5.79,13.49 5.79,12.47
N$15  (via drill 0.3 pad 0.64)
  Top 0.203: 13.1,12.15 Q2.3
  Top 0.305: Q2.3 13.28,12.48 | v13.1,11.45 13.1,12.15
  Top 0.406: 13.28,12.48 v13.28,16.01
  Top 0.61: D1.- v7.76,3.07
  Bottom 0.254: v13.28,16.01 13.3,16.03
  Bottom 0.305: v13.1,11.45 13.1,4.79 11.38,3.07 v7.76,3.07
  Bottom 0.813: 13.3,16.03 U2.1
N$16
  Top 0.203: U2.2 16.48,18.95 17.8,18.95 18.56,19.71 19.64,19.71 arc90 R2.1
N$17
  Top 0.203: U2.3 18.73,19.2 20.53,19.2 R4.1
N$26
  Top 0.203: R15.2 17.6,13.97 R16.2
  Top 0.254: R15.2 17.6,12.51 Q5.1
N$27
  Top 0.203: J1.1 8.33,37.02 R12.1
N$29
  pour Top (no thermals): 30.85,33.04 31.38,33.04 31.38,31.98 31.74,31.62 31.74,29.21 31,28.47 30.62,28.47 30.44,28.65 30.44,31.52 30.85,31.93
N$31
  Top 0.254: U3.17 14.68,24.96 C13.2 15.31,23.31 16.71,21.91 X1.1
N$32
  Top 0.254: U3.16 14.18,24.71 C14.2 13.79,23.31 12.39,21.91 X1.2
N$33
  Top 0.203: R18.2 6.49,30.86 TX.-
N$34  (via drill 0.3 pad 0.64)
  Top 0.203: R24.2 21.73,26.55 21.73,25.68 21.35,25.3 v20.08,25.3 | RX.- 9.77,33.58 v9.92,33.43
  Bottom 0.203: v20.08,25.3 19.83,25.3 18.43,26.69 18.43,34.57 17.67,35.33 16.02,35.33 15.38,35.97 12.46,35.97 v9.92,33.43
N$35
  Top 0.254: R30.1 28.01,12.39 27.96,12.34 28.1,12.34 Q7.1
N$37  (via drill 0.3 pad 0.64)
  Top 0.203: R13.1 v9.73,10.86 | U3.4 10.2,31.67 v9.92,31.39
  Bottom 0.203: v9.92,31.39 9.22,30.69 9.22,24.83 10.49,23.56 10.49,11.62 v9.73,10.86
N$38  (via drill 0.3 pad 0.64)
  Top 0.203: R14.1 v9.73,12.38 | U3.3 10.16,32.17 v9.92,32.41
  Bottom 0.203: v9.92,32.41 8.84,31.32 8.84,24.58 10.11,23.31 10.11,12.76 v9.73,12.38
N$39
  Top 0.406: R11.1 C18.1 R8.1 28.87,35.5 U1.5
N$40
  Top 0.305: R27.2 26.49,6.92 USER.2
N$41
  Top 0.406: R20.1 20.9,8.07 22.04,6.92 CHAR.2
N$42
  Top 0.406: R21.1 21.79,9.59 21.79,8.32 23.19,6.92 23.19,2.35 CHAR.1
N$43
  Top 0.254: R28.2 25.16,7.87 25.16,3.17 USER.1
N$44
  Top 0.305: R27.1 28.01,9.59 Q7.3
N$45
  Top 0.203: R28.1 22.81,9.59 Q8.3
N$46
  Top 0.254: Q8.1 24.46,14.9 R31.2
N$47
  Top 0.406: R11.2 C18.2
  Top 0.61: C18.2 27.57,32.58 27.57,29.79 L1.2 27.88,27 C3.2
  Top 0.813: C3.2 C4.2 28.9,24.07 L2.1
PAD  (via drill 0.3 pad 0.64)
  Top 0.406: U4.HEAT 38.17,22.04 v38.17,21.59
  other vias: 39.44,22.48 38.17,22.48 39.44,21.59
  pour Bottom: 40.59,24.45 40.59,20.38 37.16,20.38 37.16,24.45
PB4/A8/D8  (via drill 0.3 pad 0.64)
  Top 0.203: U3.28 19.38,30.67 19.67,30.97 21.11,30.97 v21.66,30.42 | J1.2 7.33,39.7 v7.38,39.65 | v25.42,36.98 26.61,38.18 33.8,38.18 D2.+
  Bottom 0.203: v7.38,39.65 9.41,37.62 24.78,37.62 v25.42,36.98 21.66,33.23 v21.66,30.42
PB5/A9/D9  (via drill 0.3 pad 0.64)
  Top 0.203: U3.29 19.24,31.17 19.5,31.43 21.79,31.43 24.08,29.15 24.08,22.16 v24.46,21.78
  Bottom 0.203: PWM.1 37.39,8.93 42.12,13.67 42.12,25.07 41.6,25.59 35.89,25.59 32.59,22.29 27.38,22.29 26.58,21.49 24.75,21.49 v24.46,21.78
PB7/D11  (via drill 0.3 pad 0.64)
  Top 0.203: U3.12 10.66,27.32 v10.49,27.5 | v21.54,13.53 22.8,14.79 R31.1
  Bottom 0.203: v10.49,27.5 10.49,24.83 11.25,24.07 11.25,13.53 11.63,13.15 21.16,13.15 v21.54,13.53
PC7/D13
  Top 0.203: 18.33,32.71 18.33,32.67 U3.32 arc-90 18.07,32.71 21.14,32.71 24.46,29.4 24.46,22.83 26.24,21.04 26.24,15.28 R30.2 26.48,15.09
PD0/SCL/D3  (via drill 0.3 pad 0.64)
  Top 0.203: U3.18 15.18,25.95 15.92,25.21 17.55,25.21 18.88,23.88 v18.88,23.14
  Bottom 0.203: I2C.1 45.2,8.91 44.02,10.1 44.02,26.06 42.58,27.5 35.25,27.5 31.95,24.19 19.93,24.19 v18.88,23.14
PD1/SDA/D2  (via drill 0.3 pad 0.64)
  Top 0.203: U3.19 15.68,26.06 16.15,25.59 17.75,25.59 19.51,23.83 19.51,22.5 v18.88,21.87
  Bottom 0.203: I2C.2 46.66,6.91 43.63,9.93 43.63,25.85 42.36,27.12 35.38,27.12 32.08,23.81 20.82,23.81 v18.88,21.87
PD2/RXI/D0
  Top 0.203: U3.20 16.18,26.27 16.47,25.97 17.95,25.97 19.96,23.96 R2.2
PD3/TXO/D1
  Top 0.203: U3.21 16.68,26.51 16.84,26.35 18.11,26.35 20.46,24 20.46,22.5 21.36,21.61 R4.2
PD4/A6/D4  (via drill 0.3 pad 0.64)
  Top 0.203: U3.25 22.76,29.17 23.31,28.62 23.31,22.86 v23,22.54
  Bottom 0.203: PWM.2 35.9,6.93 42.49,13.53 42.49,25.25 41.77,25.97 35.76,25.97 32.46,22.67 26.87,22.67 26.2,22 25.42,22 24.87,22.54 v23,22.54
PD5/TXLED
  Top 0.203: U3.22 17.74,27.32 18.62,26.44 20.1,26.44 R24.1
PD6/A11/D12  (via drill 0.3 pad 0.64)
  Top 0.203: U3.26 20.28,29.67 v20.46,29.85
  Top 0.254: U5.4 1.66,26.54 v1.72,26.61
  Bottom 0.203: v20.46,29.85 19.83,30.48 19.83,34.95 17.54,37.24 8.4,37.24 4.97,33.81 4.97,27.96 3.83,26.82 1.94,26.82 v1.72,26.61
  Bottom 0.305: S_OUT.T 2.36,25.04 U5.4 1.66,26.54 v1.72,26.61
PD6/D5  (via drill 0.3 pad 0.64)
  Top 0.203: U3.31 20.73,32.17 v20.84,32.07 | v24.4,36.98 25.96,38.55 32.19,38.55 D4.+
  Bottom 0.203: v24.4,36.98 20.84,33.42 v20.84,32.07
PD7/A7/D6
  Top 0.203: U3.27 19.51,30.17 19.89,30.54 20.65,30.54 21.66,29.53 23.06,29.53 23.7,28.89 23.7,19.89 22.24,18.44 22.24,17.15 20.57,15.48 20.15,15.48 | 17.61,15.45 R16.1 19.93,15.48 | 20.15,15.48 20.15,6.68 18.87,5.4 D5.+ | 19.93,15.48 20.15,15.48 | 19.93,15.48 20.14,15.26 20.34,15.45
PE6/D7  (via drill 0.3 pad 0.64)
  Top 0.203: v33.22,18.35 33.22,17.59 R34.1 33.47,17.46 33.6,17.34 33.6,16.83 34.11,16.32 34.36,16.32 R33.2 | U3.1 11.38,33.22 11.38,33.7 9.64,35.43 9.64,36.45 10.56,37.36 10.56,37.97 11,38.42 21.37,38.42 22.81,36.98 22.81,33.97 26.36,30.42 26.36,27.65 27,27.02 27,19.95 27.46,19.5 32.33,19.5 v32.71,19.88
  Top 0.254: R33.2 34.87,14.29 Q9.1
  Bottom 0.254: v32.71,19.88 33.22,19.37 v33.22,18.35
PF1/A4  (via drill 0.3 pad 0.64)
  Top 0.203: U3.40 14.18,35.01 v14.05,35.14 | v12.02,16.28 12.72,15.58 12.72,13.36 12.46,13.11 Q2.1 12.46,8.78 R9.2
  Bottom 0.203: v12.02,16.28 11.64,16.66 11.64,24.53 11.12,25.04 11.12,27.96 10.61,28.47 10.61,33.45 12.31,35.14 v14.05,35.14
PF4/A3
  Top 0.203: U3.39 14.68,36.71 16.01,38.04 21.17,38.04 22.43,36.78 22.43,33.72 25.98,30.16 25.98,27.53 26.62,26.89 26.62,19.75 27.25,19.11 33.47,19.11 34.11,18.48 34.11,16.99 34.39,16.7 35.63,16.7 R35.1
PF5/A2  (via drill 0.3 pad 0.64)
  Top 0.203: U3.38 15.18,36.65 16.18,37.66 20.97,37.66 22.04,36.58 22.04,33.53 25.6,29.97 25.6,26.92 v25.98,26.54 | v40.08,31.62 R26.1
  Top 0.254: R23.2 R26.1
  Bottom 0.203: v40.08,31.62 40.08,28.77 39.57,28.26 35,28.26 32.84,26.1 26.43,26.1 v25.98,26.54
PF6/A1  (via drill 0.3 pad 0.64)
  Top 0.203: 15.66,34.02 15.66,36.53 16.4,37.28 20.77,37.28 21.66,36.38 21.66,33.34 25.22,29.78 25.22,23.97 25.85,23.33 v25.85,22.61 | 15.66,34.02 U3.37 15.66,34.02
  Bottom 0.203: ADC.2 40.46,6.92 39.31,8.08 39.31,9.83 42.87,13.4 42.87,25.44 41.96,26.35 35.63,26.35 32.33,23.05 26.3,23.05 v25.85,22.61
PF7/A0  (via drill 0.3 pad 0.64)
  Top 0.203: U3.36 16.18,35.14 16.03,35.29 16.03,36.37 16.55,36.89 20.56,36.89 21.28,36.18 21.28,33.15 24.84,29.59 24.84,23.43 v25.09,23.18
  Bottom 0.203: ADC.1 40.46,10.48 43.25,13.27 43.25,25.64 42.16,26.73 35.51,26.73 32.2,23.43 25.6,23.43 25.35,23.18 v25.09,23.18
POWER_IN
  Top 0.203: R1.2 35,24.76
  Top 0.254: Q4.2 35,24.7 35,24.76 35,26.48 Q1.2 35.09,26.57 | D7.1 35.96,29.88 35.45,29.36 35.45,26.69 35.32,26.57 35.09,26.57 | 34.94,26.57 35.09,26.57
POWER_OUT  (via drill 0.3)
  Top 0.203: Q1.3 34.24,28.66
  Top 0.254: 34.17,28.8 34.24,28.73 34.24,28.66
  Top 0.305: U1.1 29.22,33.55 30.37,34.7 | 30.37,34.7 31.12,34.7 U1.4 | 30.37,34.7 31,35.33 31.13,35.33 31.26,35.33 30.75,34.82
  Top 0.406: 34.17,28.64 Q1.3 34.24,28.8 32.27,30.76 32.27,34.26 31.79,34.75 | 31.12,37.09 C7.2 | U1.4 | U1.4 | U1.4 31.12,34.75 31.79,34.75 | 31.79,34.75 31.2,35.33 31.13,35.33
  Top 0.61: 31.12,37.09 v31.12,36.09 U1.4
  Bottom 0.203: v31.12,36.09 32.46,34.76 44.08,34.76 45.41,33.43 T_5V.T
RESET  (via drill 0.3 pad 0.64)
  Top 0.203: U3.13 12.68,26.65 12.47,26.44 11.67,26.44 11.29,26.82 9.79,26.82 8.1,28.51 v7.82,28.51 6.91,28.51 6.11,27.71 2.65,27.71 J4.3 | v12.72,19.33 10.71,19.33 10.18,19.87 10.18,22.63 8.52,24.28 8.52,25.01 R29.1 7.69,26.73 v7.44,26.99 | R3.2 v1.92,34.76
  Top 0.61: RST.A1 41.36,28.12 v41.22,28.26
  Bottom 0.203: v41.22,28.26 40.84,27.88 35.13,27.88 32.97,25.72 32.95,25.72 31.83,24.6 18.88,24.6 18.18,23.9 18.18,20.77 16.74,19.33 v12.72,19.33 | v1.92,34.76 2.75,33.93 2.75,29.66 J4.3
  Bottom 0.254: v7.82,28.51 7.44,28.13 v7.44,26.99
USB_IN  (via drill 0.3 pad 0.64)
  Top 0.203: 15,5.34 D6.+ | U3.7 9.97,30.17 v9.92,30.12 | C16.1 9.37,15.24 9.37,15.01
  Top 0.254: R22.2 10.61,9.35 11.19,9.93 11.19,11.71 11.32,11.84 v11.32,12.38 v11.31,12.38
  Top 0.305: U4.4 38.06,25.61 D7.2 | D6.+ 14.24,4.58 v14.24,4.41
  Top 0.406: L3.2 7.57,16.85 | 9.41,15.01 9.37,15.01
  Top 0.61: C15.1 10.68,15.24 | 10.68,15.24 C16.1 9.26,15.33 9.16,15.33 7.64,16.85 7.57,16.85 | L3.2 5.42,16.85 D8.2 | v11.31,12.38 11.31,14.61 10.68,15.24
  Top 0.813: v36.4,21.91 36.4,24.48 D7.2
  Bottom 0.203: 13.86,12.34 13.77,12.34 13.73,12.38
  Bottom 0.254: v9.92,30.12 9.73,29.93 9.73,24.96 10.87,23.81 10.87,12.71 11.19,12.38 | 11.12,12.38 11.19,12.38 | 11.19,12.38 v11.31,12.38
  Bottom 0.305: 13.86,12.34 13.86,11.96 | 13.86,11.96 13.86,4.79 v14.24,4.41 | 13.86,11.96 13.6,12.22 | 13.86,11.96 14.11,12.22
  Bottom 0.813: v36.4,21.91 36.4,18.48 30.3,12.38 13.73,12.38 v11.31,12.38

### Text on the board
tPlace: - | + | V0.91 change note: / add diodes D4 / add MOSFET Q10 / add 3pin connector / change buzzer size / change POWER LED position / change DC-DC inductance size / change reset button size / change switch size / 2013/1/5 Bruce / change reset cirvuit del reset LED / fix bug / 2013/2/20
bPlace: Atom Node | v1.0 02/20/2013 | by Seeed Studio | www.seeedstudio.com
bNames: Bat- | Bat+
